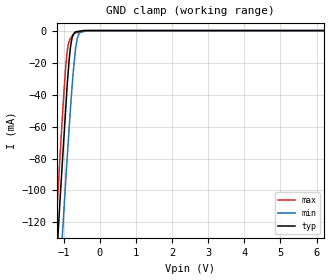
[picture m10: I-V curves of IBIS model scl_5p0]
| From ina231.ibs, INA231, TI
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|   scl_5p0 Model
[Model]   scl_5p0
Model_type   Input
Vinl = 0.4
Vinh = 1.4
|   typ   min   max
|   (nom PVT)   (fast PVT)   (slow PVT)
|C_comp from frequency sweep method (F=100KHz)
|Average
|C_comp   1.942e-12   1.542e-12   2.390e-12
|C_comp from LC tank measurement(L=1nH)
|Average
|Resonant Frequency(Hz)   5.430e+09   5.490e+09   5.410e+09
C_comp   8.599e-13   8.413e-13   8.663e-13
| Where nom  PVT is Nominal Process, 5V, 27C
|   Fast PVT is Strong Process,  5.5V, -40C
|   Slow PVT is Weak Process,   4.5V, 125C
[Voltage Range]   5   4.5   5.5
|Ambient Temperature   25   150   -65
|Junction Temperature
[Temperature Range]   27   125   -40
[Power Clamp Reference]   5   4.5   5.5
[GND Clamp Reference]   0   0   0
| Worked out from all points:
|   GND clamp passes 1 mA (typ) near -0.68 V on its own axis
[GND Clamp]
|   Voltage   I(typ)   I(min)   I(max)
-5V       -1.74A     -1.75A     -1.742A
-1.221V   -152.7mA   -198.2mA   -125.7mA
-1.183V   -137.7mA   -183.5mA   -110.7mA
-1.14V    -120.3mA   -166.9mA   -93.34mA
-1.03V    -79.59mA   -125.2mA   -51.31mA
-951.5mV  -51.05mA   -96.15mA   -24.5mA
-907.5mV  -35.15mA   -80.36mA   -13.51mA
-800mV    -8.092mA   -44.33mA   -4.367mA
-670mV    -759.1uA   -11.05mA   -1.561mA
-567mV    -427.7uA   -1.469mA   -771.1uA
-351mV    -2.343uA   -6.884uA   -6.043uA
10V       0A         0A         0A
[POWER Clamp]
|   Voltage   I(typ)   I(min)   I(max)
-5V       0A         0A         0A
-5V       0A         0A         0A
10V       0A         0A         0A
